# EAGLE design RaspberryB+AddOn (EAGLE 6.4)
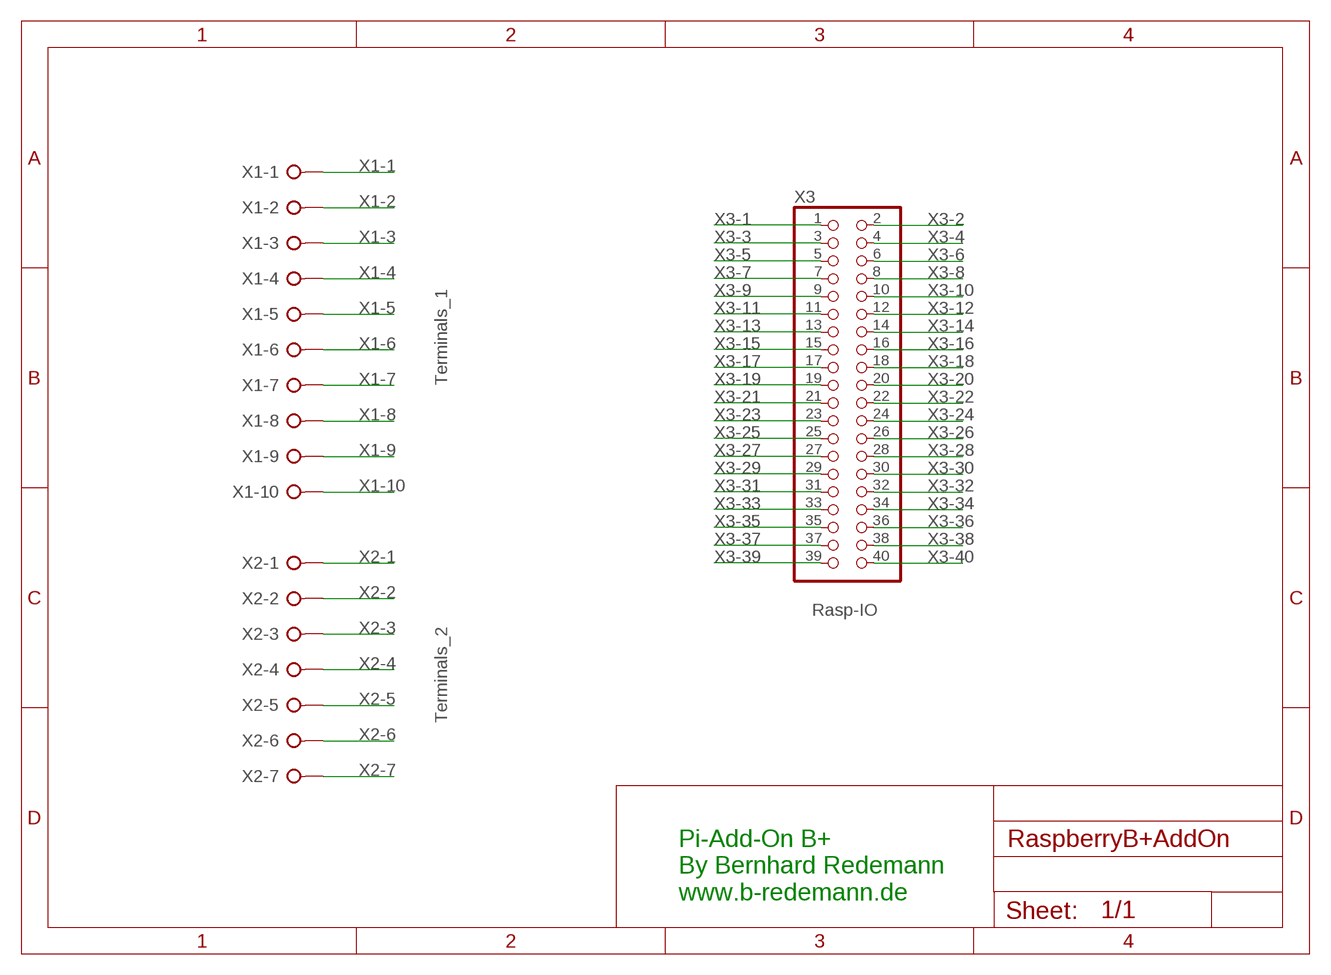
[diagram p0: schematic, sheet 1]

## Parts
X1  Terminals_1  W237-10P  [W237-10P]
X2  Terminals_2  W237-07P  [W237-7P]
X3  Rasp-IO  PINHD-2X20  [2X20]

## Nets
X1-1: X1.1
X1-2: X1.2
X1-3: X1.3
X1-4: X1.4
X1-5: X1.5
X1-6: X1.6
X1-7: X1.7
X1-8: X1.8
X1-9: X1.9
X1-10: X1.10
X2-1: X2.1
X2-2: X2.2
X2-3: X2.3
X2-4: X2.4
X2-5: X2.5
X2-6: X2.6
X2-7: X2.7
X3-1: X3.1
X3-2: X3.2
X3-3: X3.3
X3-4: X3.4
X3-5: X3.5
X3-6: X3.6
X3-7: X3.7
X3-8: X3.8
X3-9: X3.9
X3-10: X3.10
X3-11: X3.11
X3-12: X3.12
X3-13: X3.13
X3-14: X3.14
X3-15: X3.15
X3-16: X3.16
X3-17: X3.17
X3-18: X3.18
X3-19: X3.19
X3-20: X3.20
X3-21: X3.21
X3-22: X3.22
X3-23: X3.23
X3-24: X3.24
X3-25: X3.25
X3-26: X3.26
X3-27: X3.27
X3-28: X3.28
X3-29: X3.29
X3-30: X3.30
X3-31: X3.31
X3-32: X3.32
X3-33: X3.33
X3-34: X3.34
X3-35: X3.35
X3-36: X3.36
X3-37: X3.37
X3-38: X3.38
X3-39: X3.39
X3-40: X3.40

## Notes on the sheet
- Pi-Add-On B+
  By Bernhard Redemann
  www.b-redemann.de

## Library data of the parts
X1 = con-wago-508:W237-10P: WAGO SREW CLAMP; OC_FARNELL: unknown; OC_NEWARK: unknown
X2 = con-wago-508:W237-07P: WAGO SREW CLAMP; OC_FARNELL: unknown; OC_NEWARK: unknown
X3 = pinhead:PINHD-2X20: PIN HEADER

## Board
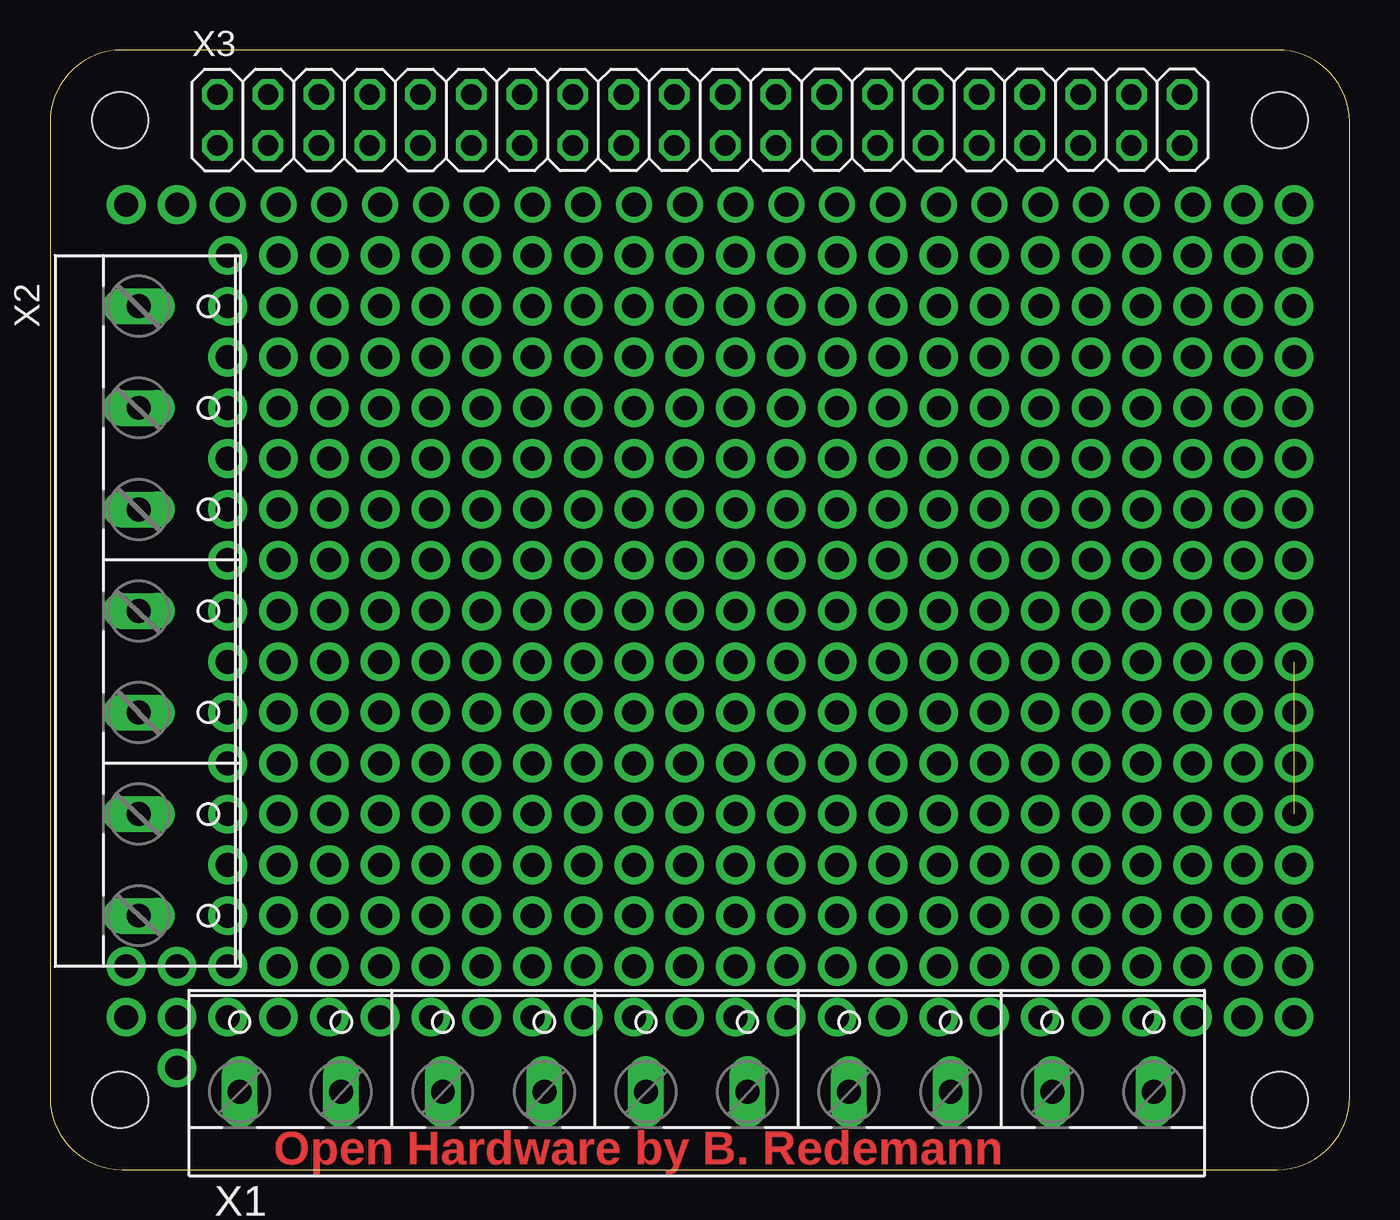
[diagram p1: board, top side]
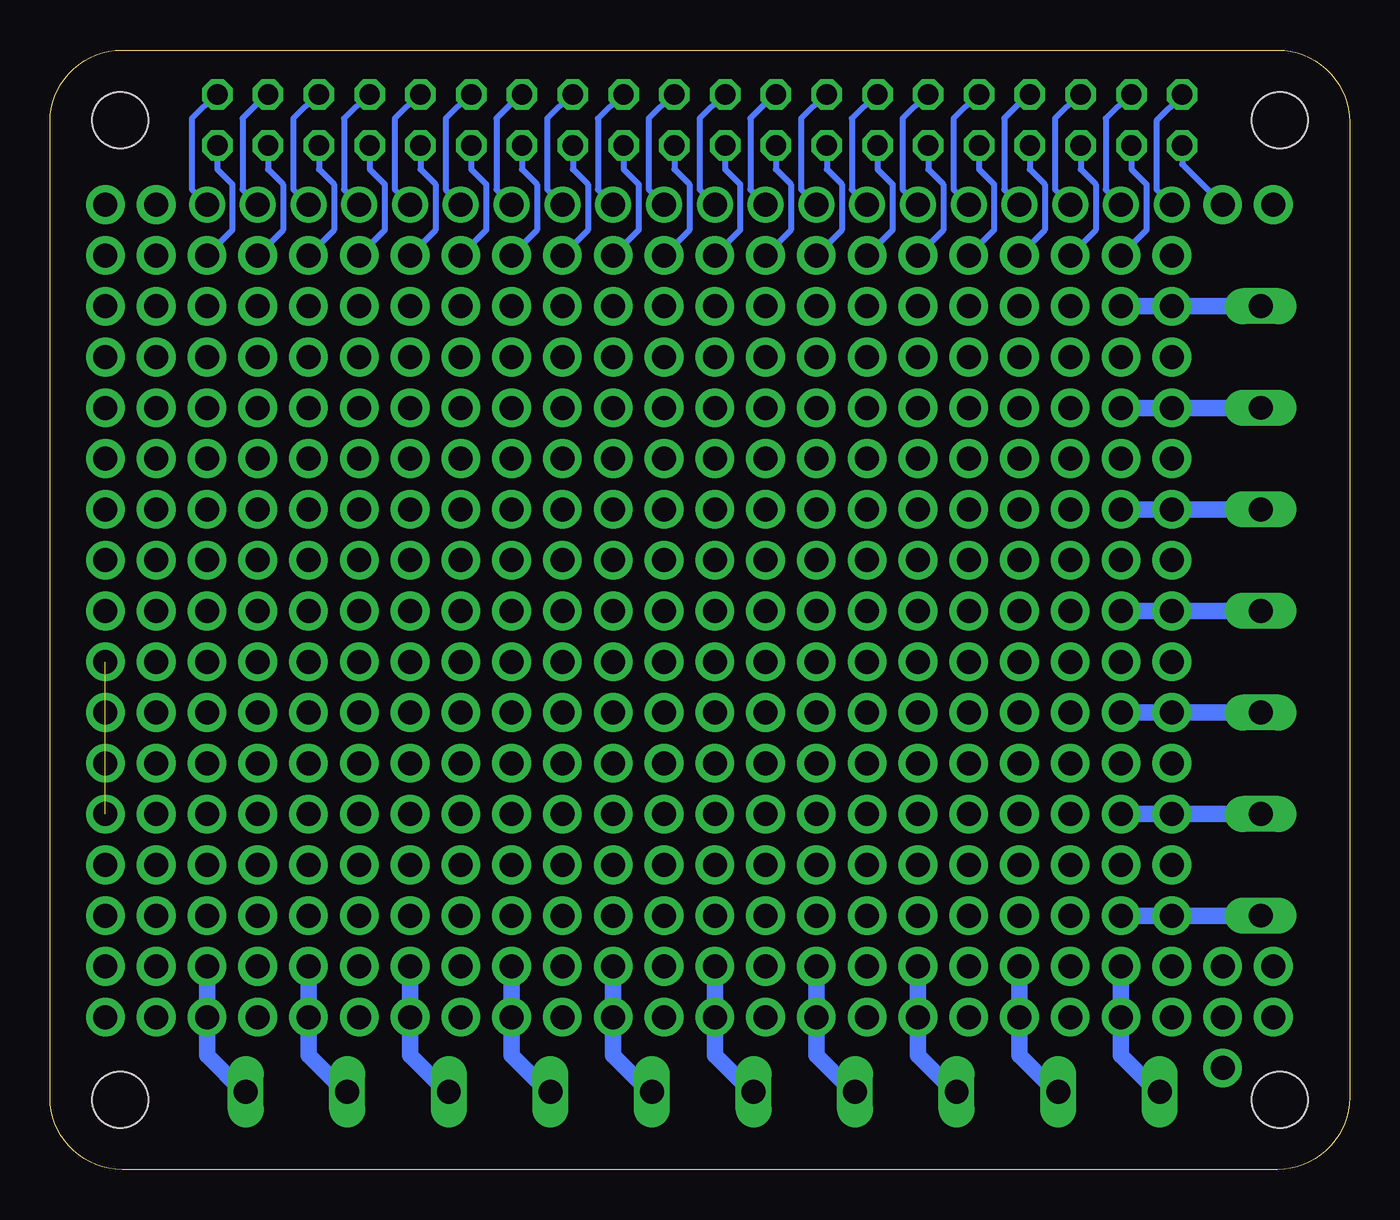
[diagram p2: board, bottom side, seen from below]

Size 65 x 56 mm. Coordinates in mm from the lower left corner, seen from the top.
Outline: 61.39,56 3.61,56 arc90 0,52.39 0,3.61 arc90 3.61,0 61.39,0 arc90 65,3.61 65,52.39 arc90 61.39,56
Copper layers (1*16): Top 0.035mm / dielectric 1.5mm / Bottom 0.035mm
Design rules "default": minimum track width 10mil, minimum drill 24mil, track to track 8mil, track to pad 8mil, pad to pad 8mil, via to via 8mil, smd to smd 8mil, copper to edge 40mil, drill to drill 8mil, minimum pad ring 10mil, minimum via ring 8mil, stop-mask expansion 4mil, vias tented up to drill 0mil, thermal gap 10mil
Holes 2.8 mm at 3.5,3.5 3.5,52.5 61.5,3.5 61.5,52.5

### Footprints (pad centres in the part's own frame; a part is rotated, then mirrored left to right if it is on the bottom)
W237-10P = drill 1.194 long: 1 -22.86,-0.635; 2 -17.78,-0.635; 3 -12.7,-0.635; 4 -7.62,-0.635; 5 -2.54,-0.635; 6 2.54,-0.635; 7 7.62,-0.635; 8 12.7,-0.635; 9 17.78,-0.635; 10 22.86,-0.635
W237-7P = drill 1.194 long: 1 -15.24,-0.635; 2 -10.16,-0.635; 3 -5.08,-0.635; 4 0,-0.635; 5 5.08,-0.635; 6 10.16,-0.635; 7 15.24,-0.635
2X20 = drill 1.016 octagon: 1 -24.13,-1.27; 2 -24.13,1.27; 3 -21.59,-1.27; 4 -21.59,1.27; 5 -19.05,-1.27; 6 -19.05,1.27; 7 -16.51,-1.27; 8 -16.51,1.27; 9 -13.97,-1.27; 10 -13.97,1.27; 11 -11.43,-1.27; 12 -11.43,1.27; 13 -8.89,-1.27; 14 -8.89,1.27; 15 -6.35,-1.27; 16 -6.35,1.27; 17 -3.81,-1.27; 18 -3.81,1.27; 19 -1.27,-1.27; 20 -1.27,1.27; 21 1.27,-1.27; 22 1.27,1.27; 23 3.81,-1.27; 24 3.81,1.27; 25 6.35,-1.27; 26 6.35,1.27; 27 8.89,-1.27; 28 8.89,1.27; 29 11.43,-1.27; 30 11.43,1.27; 31 13.97,-1.27; 32 13.97,1.27; 33 16.51,-1.27; 34 16.51,1.27; 35 19.05,-1.27; 36 19.05,1.27; 37 21.59,-1.27; 38 21.59,1.27; 39 24.13,-1.27; 40 24.13,1.27

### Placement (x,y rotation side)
X1  32.35,4.53 0 top
X2  5.08,27.94 270 top
X3  32.5,52.5 0 top

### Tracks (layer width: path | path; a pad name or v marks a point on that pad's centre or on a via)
N$1  (via drill 1.2 pad 1.93)
  other vias: 3.81,48.26
N$23  (via drill 1.2 pad 1.93)
  other vias: 59.69,48.26
N$24  (via drill 1.2 pad 1.93)
  other vias: 62.23,48.26
N$25  (via drill 1.2 pad 1.93)
  other vias: 62.23,45.72
N$26  (via drill 1.2 pad 1.93)
  other vias: 59.69,45.72
N$54  (via drill 1.2 pad 1.93)
  other vias: 8.89,45.72
N$55  (via drill 1.2 pad 1.93)
  other vias: 13.97,43.18
N$56  (via drill 1.2 pad 1.93)
  other vias: 16.51,43.18
N$57  (via drill 1.2 pad 1.93)
  other vias: 19.05,43.18
N$58  (via drill 1.2 pad 1.93)
  other vias: 21.59,43.18
N$59  (via drill 1.2 pad 1.93)
  other vias: 24.13,43.18
N$60  (via drill 1.2 pad 1.93)
  other vias: 26.67,43.18
N$61  (via drill 1.2 pad 1.93)
  other vias: 29.21,43.18
N$62  (via drill 1.2 pad 1.93)
  other vias: 31.75,43.18
N$63  (via drill 1.2 pad 1.93)
  other vias: 34.29,43.18
N$64  (via drill 1.2 pad 1.93)
  other vias: 36.83,43.18
N$65  (via drill 1.2 pad 1.93)
  other vias: 39.37,43.18
N$66  (via drill 1.2 pad 1.93)
  other vias: 41.91,43.18
N$67  (via drill 1.2 pad 1.93)
  other vias: 44.45,43.18
N$68  (via drill 1.2 pad 1.93)
  other vias: 46.99,43.18
N$69  (via drill 1.2 pad 1.93)
  other vias: 49.53,43.18
N$70  (via drill 1.2 pad 1.93)
  other vias: 52.07,43.18
N$71  (via drill 1.2 pad 1.93)
  other vias: 54.61,43.18
N$72  (via drill 1.2 pad 1.93)
  other vias: 57.15,43.18
N$73  (via drill 1.2 pad 1.93)
  other vias: 59.69,43.18
N$74  (via drill 1.2 pad 1.93)
  other vias: 62.23,43.18
N$75  (via drill 1.2 pad 1.93)
  other vias: 62.23,40.64
N$76  (via drill 1.2 pad 1.93)
  other vias: 62.23,38.1
N$77  (via drill 1.2 pad 1.93)
  other vias: 59.69,40.64
N$78  (via drill 1.2 pad 1.93)
  other vias: 59.69,38.1
N$79  (via drill 1.2 pad 1.93)
  other vias: 57.15,40.64
N$80  (via drill 1.2 pad 1.93)
  other vias: 57.15,38.1
N$81  (via drill 1.2 pad 1.93)
  other vias: 54.61,40.64
N$82  (via drill 1.2 pad 1.93)
  other vias: 54.61,38.1
N$83  (via drill 1.2 pad 1.93)
  other vias: 52.07,40.64
N$84  (via drill 1.2 pad 1.93)
  other vias: 52.07,38.1
N$85  (via drill 1.2 pad 1.93)
  other vias: 49.53,40.64
N$86  (via drill 1.2 pad 1.93)
  other vias: 49.53,38.1
N$87  (via drill 1.2 pad 1.93)
  other vias: 46.99,40.64
N$88  (via drill 1.2 pad 1.93)
  other vias: 46.99,38.1
N$89  (via drill 1.2 pad 1.93)
  other vias: 44.45,40.64
N$90  (via drill 1.2 pad 1.93)
  other vias: 44.45,38.1
N$91  (via drill 1.2 pad 1.93)
  other vias: 41.91,40.64
N$92  (via drill 1.2 pad 1.93)
  other vias: 41.91,38.1
N$93  (via drill 1.2 pad 1.93)
  other vias: 39.37,40.64
N$94  (via drill 1.2 pad 1.93)
  other vias: 39.37,38.1
N$95  (via drill 1.2 pad 1.93)
  other vias: 36.83,40.64
N$96  (via drill 1.2 pad 1.93)
  other vias: 36.83,38.1
N$97  (via drill 1.2 pad 1.93)
  other vias: 34.29,40.64
N$98  (via drill 1.2 pad 1.93)
  other vias: 34.29,38.1
N$99  (via drill 1.2 pad 1.93)
  other vias: 31.75,40.64
N$100  (via drill 1.2 pad 1.93)
  other vias: 31.75,38.1
N$101  (via drill 1.2 pad 1.93)
  other vias: 29.21,40.64
N$102  (via drill 1.2 pad 1.93)
  other vias: 29.21,38.1
N$103  (via drill 1.2 pad 1.93)
  other vias: 26.67,40.64
N$104  (via drill 1.2 pad 1.93)
  other vias: 26.67,38.1
N$105  (via drill 1.2 pad 1.93)
  other vias: 24.13,40.64
N$106  (via drill 1.2 pad 1.93)
  other vias: 24.13,38.1
N$107  (via drill 1.2 pad 1.93)
  other vias: 21.59,40.64
N$108  (via drill 1.2 pad 1.93)
  other vias: 21.59,38.1
N$109  (via drill 1.2 pad 1.93)
  other vias: 19.05,40.64
N$110  (via drill 1.2 pad 1.93)
  other vias: 19.05,38.1
N$111  (via drill 1.2 pad 1.93)
  other vias: 16.51,40.64
N$112  (via drill 1.2 pad 1.93)
  other vias: 16.51,38.1
N$113  (via drill 1.2 pad 1.93)
  other vias: 13.97,40.64
N$114  (via drill 1.2 pad 1.93)
  other vias: 13.97,38.1
N$116  (via drill 1.2 pad 1.93)
  other vias: 8.89,40.64
N$118  (via drill 1.2 pad 1.93)
  other vias: 11.43,40.64
N$125  (via drill 1.2 pad 1.93)
  other vias: 13.97,35.56
N$126  (via drill 1.2 pad 1.93)
  other vias: 16.51,35.56
N$127  (via drill 1.2 pad 1.93)
  other vias: 19.05,35.56
N$128  (via drill 1.2 pad 1.93)
  other vias: 21.59,35.56
N$129  (via drill 1.2 pad 1.93)
  other vias: 24.13,35.56
N$130  (via drill 1.2 pad 1.93)
  other vias: 26.67,35.56
N$131  (via drill 1.2 pad 1.93)
  other vias: 29.21,35.56
N$132  (via drill 1.2 pad 1.93)
  other vias: 31.75,35.56
N$133  (via drill 1.2 pad 1.93)
  other vias: 34.29,35.56
N$134  (via drill 1.2 pad 1.93)
  other vias: 36.83,35.56
N$135  (via drill 1.2 pad 1.93)
  other vias: 39.37,35.56
N$136  (via drill 1.2 pad 1.93)
  other vias: 41.91,35.56
N$137  (via drill 1.2 pad 1.93)
  other vias: 44.45,35.56
N$138  (via drill 1.2 pad 1.93)
  other vias: 46.99,35.56
N$139  (via drill 1.2 pad 1.93)
  other vias: 49.53,35.56
N$140  (via drill 1.2 pad 1.93)
  other vias: 52.07,35.56
N$141  (via drill 1.2 pad 1.93)
  other vias: 54.61,35.56
N$142  (via drill 1.2 pad 1.93)
  other vias: 57.15,35.56
N$143  (via drill 1.2 pad 1.93)
  other vias: 59.69,35.56
N$144  (via drill 1.2 pad 1.93)
  other vias: 62.23,35.56
N$145  (via drill 1.2 pad 1.93)
  other vias: 62.23,33.02
N$146  (via drill 1.2 pad 1.93)
  other vias: 62.23,30.48
N$147  (via drill 1.2 pad 1.93)
  other vias: 62.23,27.94
N$150  (via drill 1.2 pad 1.93)
  other vias: 8.89,35.56
N$151  (via drill 1.2 pad 1.93)
  other vias: 11.43,35.56
N$152  (via drill 1.2 pad 1.93)
  other vias: 13.97,33.02
N$153  (via drill 1.2 pad 1.93)
  other vias: 16.51,33.02
N$154  (via drill 1.2 pad 1.93)
  other vias: 19.05,33.02
N$155  (via drill 1.2 pad 1.93)
  other vias: 21.59,33.02
N$156  (via drill 1.2 pad 1.93)
  other vias: 24.13,33.02
N$157  (via drill 1.2 pad 1.93)
  other vias: 26.67,33.02
N$158  (via drill 1.2 pad 1.93)
  other vias: 29.21,33.02
N$159  (via drill 1.2 pad 1.93)
  other vias: 31.75,33.02
N$160  (via drill 1.2 pad 1.93)
  other vias: 34.29,33.02
N$161  (via drill 1.2 pad 1.93)
  other vias: 36.83,33.02
N$162  (via drill 1.2 pad 1.93)
  other vias: 39.37,33.02
N$163  (via drill 1.2 pad 1.93)
  other vias: 41.91,33.02
N$164  (via drill 1.2 pad 1.93)
  other vias: 44.45,33.02
N$165  (via drill 1.2 pad 1.93)
  other vias: 46.99,33.02
N$166  (via drill 1.2 pad 1.93)
  other vias: 49.53,33.02
N$167  (via drill 1.2 pad 1.93)
  other vias: 52.07,33.02
N$168  (via drill 1.2 pad 1.93)
  other vias: 54.61,33.02
N$169  (via drill 1.2 pad 1.93)
  other vias: 57.15,33.02
N$170  (via drill 1.2 pad 1.93)
  other vias: 59.69,33.02
N$171  (via drill 1.2 pad 1.93)
  other vias: 59.69,30.48
N$172  (via drill 1.2 pad 1.93)
  other vias: 57.15,30.48
N$173  (via drill 1.2 pad 1.93)
  other vias: 54.61,30.48
N$174  (via drill 1.2 pad 1.93)
  other vias: 52.07,30.48
N$175  (via drill 1.2 pad 1.93)
  other vias: 49.53,30.48
N$176  (via drill 1.2 pad 1.93)
  other vias: 46.99,30.48
N$177  (via drill 1.2 pad 1.93)
  other vias: 44.45,30.48
N$178  (via drill 1.2 pad 1.93)
  other vias: 41.91,30.48
N$179  (via drill 1.2 pad 1.93)
  other vias: 39.37,30.48
N$180  (via drill 1.2 pad 1.93)
  other vias: 36.83,30.48
N$181  (via drill 1.2 pad 1.93)
  other vias: 34.29,30.48
N$182  (via drill 1.2 pad 1.93)
  other vias: 31.75,30.48
N$183  (via drill 1.2 pad 1.93)
  other vias: 29.21,30.48
N$184  (via drill 1.2 pad 1.93)
  other vias: 26.67,30.48
N$185  (via drill 1.2 pad 1.93)
  other vias: 24.13,30.48
N$186  (via drill 1.2 pad 1.93)
  other vias: 21.59,30.48
N$187  (via drill 1.2 pad 1.93)
  other vias: 19.05,30.48
N$188  (via drill 1.2 pad 1.93)
  other vias: 16.51,30.48
N$189  (via drill 1.2 pad 1.93)
  other vias: 13.97,30.48
N$198  (via drill 1.2 pad 1.93)
  other vias: 8.89,30.48
N$199  (via drill 1.2 pad 1.93)
  other vias: 11.43,30.48
N$200  (via drill 1.2 pad 1.93)
  other vias: 13.97,27.94
N$201  (via drill 1.2 pad 1.93)
  other vias: 16.51,27.94
N$202  (via drill 1.2 pad 1.93)
  other vias: 19.05,27.94
N$203  (via drill 1.2 pad 1.93)
  other vias: 21.59,27.94
N$204  (via drill 1.2 pad 1.93)
  other vias: 24.13,27.94
N$205  (via drill 1.2 pad 1.93)
  other vias: 26.67,27.94
N$206  (via drill 1.2 pad 1.93)
  other vias: 29.21,27.94
N$207  (via drill 1.2 pad 1.93)
  other vias: 31.75,27.94
N$208  (via drill 1.2 pad 1.93)
  other vias: 34.29,27.94
N$209  (via drill 1.2 pad 1.93)
  other vias: 36.83,27.94
N$210  (via drill 1.2 pad 1.93)
  other vias: 39.37,27.94
N$211  (via drill 1.2 pad 1.93)
  other vias: 41.91,27.94
N$212  (via drill 1.2 pad 1.93)
  other vias: 44.45,27.94
N$213  (via drill 1.2 pad 1.93)
  other vias: 46.99,27.94
N$214  (via drill 1.2 pad 1.93)
  other vias: 49.53,27.94
N$215  (via drill 1.2 pad 1.93)
  other vias: 52.07,27.94
N$216  (via drill 1.2 pad 1.93)
  other vias: 54.61,27.94
N$217  (via drill 1.2 pad 1.93)
  other vias: 57.15,27.94
N$218  (via drill 1.2 pad 1.93)
  other vias: 59.69,27.94
N$219  (via drill 1.2 pad 1.93)
  other vias: 59.69,25.4
N$220  (via drill 1.2 pad 1.93)
  other vias: 59.69,22.86
N$221  (via drill 1.2 pad 1.93)
  other vias: 57.15,25.4
N$222  (via drill 1.2 pad 1.93)
  other vias: 57.15,22.86
N$223  (via drill 1.2 pad 1.93)
  other vias: 54.61,25.4
N$224  (via drill 1.2 pad 1.93)
  other vias: 54.61,22.86
N$225  (via drill 1.2 pad 1.93)
  other vias: 52.07,25.4
N$226  (via drill 1.2 pad 1.93)
  other vias: 52.07,22.86
N$227  (via drill 1.2 pad 1.93)
  other vias: 49.53,25.4
N$228  (via drill 1.2 pad 1.93)
  other vias: 49.53,22.86
N$229  (via drill 1.2 pad 1.93)
  other vias: 46.99,25.4
N$230  (via drill 1.2 pad 1.93)
  other vias: 46.99,22.86
N$231  (via drill 1.2 pad 1.93)
  other vias: 44.45,25.4
N$232  (via drill 1.2 pad 1.93)
  other vias: 44.45,22.86
N$233  (via drill 1.2 pad 1.93)
  other vias: 41.91,25.4
N$234  (via drill 1.2 pad 1.93)
  other vias: 41.91,22.86
N$235  (via drill 1.2 pad 1.93)
  other vias: 39.37,25.4
N$236  (via drill 1.2 pad 1.93)
  other vias: 39.37,22.86
N$237  (via drill 1.2 pad 1.93)
  other vias: 36.83,25.4
N$238  (via drill 1.2 pad 1.93)
  other vias: 36.83,22.86
N$239  (via drill 1.2 pad 1.93)
  other vias: 34.29,25.4
N$240  (via drill 1.2 pad 1.93)
  other vias: 34.29,22.86
N$241  (via drill 1.2 pad 1.93)
  other vias: 31.75,25.4
N$242  (via drill 1.2 pad 1.93)
  other vias: 31.75,22.86
N$243  (via drill 1.2 pad 1.93)
  other vias: 29.21,25.4
N$244  (via drill 1.2 pad 1.93)
  other vias: 29.21,22.86
N$245  (via drill 1.2 pad 1.93)
  other vias: 26.67,25.4
N$246  (via drill 1.2 pad 1.93)
  other vias: 26.67,22.86
N$247  (via drill 1.2 pad 1.93)
  other vias: 24.13,25.4
N$248  (via drill 1.2 pad 1.93)
  other vias: 24.13,22.86
N$249  (via drill 1.2 pad 1.93)
  other vias: 21.59,25.4
N$250  (via drill 1.2 pad 1.93)
  other vias: 21.59,22.86
N$251  (via drill 1.2 pad 1.93)
  other vias: 19.05,25.4
N$252  (via drill 1.2 pad 1.93)
  other vias: 19.05,22.86
N$253  (via drill 1.2 pad 1.93)
  other vias: 16.51,25.4
N$254  (via drill 1.2 pad 1.93)
  other vias: 16.51,22.86
N$255  (via drill 1.2 pad 1.93)
  other vias: 13.97,25.4
N$256  (via drill 1.2 pad 1.93)
  other vias: 13.97,22.86
N$258  (via drill 1.2 pad 1.93)
  other vias: 11.43,25.4
N$260  (via drill 1.2 pad 1.93)
  other vias: 8.89,25.4
N$267  (via drill 1.2 pad 1.93)
  other vias: 13.97,20.32
N$268  (via drill 1.2 pad 1.93)
  other vias: 16.51,20.32
N$269  (via drill 1.2 pad 1.93)
  other vias: 19.05,20.32
N$270  (via drill 1.2 pad 1.93)
  other vias: 21.59,20.32
N$271  (via drill 1.2 pad 1.93)
  other vias: 24.13,20.32
N$272  (via drill 1.2 pad 1.93)
  other vias: 26.67,20.32
N$273  (via drill 1.2 pad 1.93)
  other vias: 29.21,20.32
N$274  (via drill 1.2 pad 1.93)
  other vias: 31.75,20.32
N$275  (via drill 1.2 pad 1.93)
  other vias: 34.29,20.32
N$276  (via drill 1.2 pad 1.93)
  other vias: 36.83,20.32
N$277  (via drill 1.2 pad 1.93)
  other vias: 39.37,20.32
N$278  (via drill 1.2 pad 1.93)
  other vias: 41.91,20.32
N$279  (via drill 1.2 pad 1.93)
  other vias: 44.45,20.32
N$280  (via drill 1.2 pad 1.93)
  other vias: 46.99,20.32
N$281  (via drill 1.2 pad 1.93)
  other vias: 49.53,20.32
N$282  (via drill 1.2 pad 1.93)
  other vias: 52.07,20.32
N$283  (via drill 1.2 pad 1.93)
  other vias: 54.61,20.32
N$284  (via drill 1.2 pad 1.93)
  other vias: 57.15,20.32
N$285  (via drill 1.2 pad 1.93)
  other vias: 59.69,20.32
N$286  (via drill 1.2 pad 1.93)  (3 unrouted)
  other vias: 62.23,17.78 62.23,20.32 62.23,22.86 62.23,25.4
N$287  (via drill 1.2 pad 1.93)
  other vias: 62.23,15.24
N$288  (via drill 1.2 pad 1.93)
  other vias: 62.23,12.7
N$291  (via drill 1.2 pad 1.93)
  other vias: 8.89,20.32
N$292  (via drill 1.2 pad 1.93)
  other vias: 11.43,20.32
N$293  (via drill 1.2 pad 1.93)
  other vias: 13.97,17.78
N$294  (via drill 1.2 pad 1.93)
  other vias: 16.51,17.78
N$295  (via drill 1.2 pad 1.93)
  other vias: 19.05,17.78
N$296  (via drill 1.2 pad 1.93)
  other vias: 21.59,17.78
N$297  (via drill 1.2 pad 1.93)
  other vias: 24.13,17.78
N$298  (via drill 1.2 pad 1.93)
  other vias: 26.67,17.78
N$299  (via drill 1.2 pad 1.93)
  other vias: 29.21,17.78
N$300  (via drill 1.2 pad 1.93)
  other vias: 31.75,17.78
N$301  (via drill 1.2 pad 1.93)
  other vias: 34.29,17.78
N$302  (via drill 1.2 pad 1.93)
  other vias: 36.83,17.78
N$303  (via drill 1.2 pad 1.93)
  other vias: 39.37,17.78
N$304  (via drill 1.2 pad 1.93)
  other vias: 41.91,17.78
N$305  (via drill 1.2 pad 1.93)
  other vias: 44.45,17.78
N$306  (via drill 1.2 pad 1.93)
  other vias: 46.99,17.78
N$307  (via drill 1.2 pad 1.93)
  other vias: 49.53,17.78
N$308  (via drill 1.2 pad 1.93)
  other vias: 52.07,17.78
N$309  (via drill 1.2 pad 1.93)
  other vias: 54.61,17.78
N$310  (via drill 1.2 pad 1.93)
  other vias: 57.15,17.78
N$311  (via drill 1.2 pad 1.93)
  other vias: 59.69,17.78
N$312  (via drill 1.2 pad 1.93)
  other vias: 59.69,15.24
N$313  (via drill 1.2 pad 1.93)
  other vias: 57.15,15.24
N$314  (via drill 1.2 pad 1.93)
  other vias: 54.61,15.24
N$315  (via drill 1.2 pad 1.93)
  other vias: 52.07,15.24
N$316  (via drill 1.2 pad 1.93)
  other vias: 49.53,15.24
N$317  (via drill 1.2 pad 1.93)
  other vias: 46.99,15.24
N$318  (via drill 1.2 pad 1.93)
  other vias: 44.45,15.24
N$319  (via drill 1.2 pad 1.93)
  other vias: 41.91,15.24
N$320  (via drill 1.2 pad 1.93)
  other vias: 39.37,15.24
N$321  (via drill 1.2 pad 1.93)
  other vias: 36.83,15.24
N$322  (via drill 1.2 pad 1.93)
  other vias: 34.29,15.24
N$323  (via drill 1.2 pad 1.93)
  other vias: 31.75,15.24
N$324  (via drill 1.2 pad 1.93)
  other vias: 29.21,15.24
N$325  (via drill 1.2 pad 1.93)
  other vias: 26.67,15.24
N$326  (via drill 1.2 pad 1.93)
  other vias: 24.13,15.24
N$327  (via drill 1.2 pad 1.93)
  other vias: 21.59,15.24
N$328  (via drill 1.2 pad 1.93)
  other vias: 19.05,15.24
N$329  (via drill 1.2 pad 1.93)
  other vias: 16.51,15.24
N$330  (via drill 1.2 pad 1.93)
  other vias: 13.97,15.24
N$336  (via drill 1.2 pad 1.93)
  other vias: 3.81,10.16
N$337  (via drill 1.2 pad 1.93)
  other vias: 6.35,10.16
N$339  (via drill 1.2 pad 1.93)
  other vias: 11.43,15.24
N$340  (via drill 1.2 pad 1.93)
  other vias: 8.89,15.24
N$341  (via drill 1.2 pad 1.93)
  other vias: 13.97,12.7
N$342  (via drill 1.2 pad 1.93)
  other vias: 16.51,12.7
N$343  (via drill 1.2 pad 1.93)
  other vias: 19.05,12.7
N$344  (via drill 1.2 pad 1.93)
  other vias: 21.59,12.7
N$345  (via drill 1.2 pad 1.93)
  other vias: 24.13,12.7
N$346  (via drill 1.2 pad 1.93)
  other vias: 26.67,12.7
N$347  (via drill 1.2 pad 1.93)
  other vias: 29.21,12.7
N$348  (via drill 1.2 pad 1.93)
  other vias: 31.75,12.7
N$349  (via drill 1.2 pad 1.93)
  other vias: 34.29,12.7
N$350  (via drill 1.2 pad 1.93)
  other vias: 36.83,12.7
N$351  (via drill 1.2 pad 1.93)
  other vias: 39.37,12.7
N$352  (via drill 1.2 pad 1.93)
  other vias: 41.91,12.7
N$353  (via drill 1.2 pad 1.93)
  other vias: 44.45,12.7
N$354  (via drill 1.2 pad 1.93)
  other vias: 46.99,12.7
N$355  (via drill 1.2 pad 1.93)
  other vias: 49.53,12.7
N$356  (via drill 1.2 pad 1.93)
  other vias: 52.07,12.7
N$357  (via drill 1.2 pad 1.93)
  other vias: 54.61,12.7
N$358  (via drill 1.2 pad 1.93)
  other vias: 57.15,12.7
N$359  (via drill 1.2 pad 1.93)
  other vias: 59.69,12.7
N$360  (via drill 1.2 pad 1.93)
  other vias: 59.69,10.16
N$361  (via drill 1.2 pad 1.93)
  other vias: 59.69,7.62
N$364  (via drill 1.2 pad 1.93)
  other vias: 54.61,10.16
N$365  (via drill 1.2 pad 1.93)
  other vias: 54.61,7.62
N$368  (via drill 1.2 pad 1.93)
  other vias: 49.53,10.16
N$369  (via drill 1.2 pad 1.93)
  other vias: 49.53,7.62
N$372  (via drill 1.2 pad 1.93)
  other vias: 44.45,10.16
N$373  (via drill 1.2 pad 1.93)
  other vias: 44.45,7.62
N$376  (via drill 1.2 pad 1.93)
  other vias: 39.37,10.16
N$377  (via drill 1.2 pad 1.93)
  other vias: 39.37,7.62
N$380  (via drill 1.2 pad 1.93)
  other vias: 34.29,10.16
N$381  (via drill 1.2 pad 1.93)
  other vias: 34.29,7.62
N$384  (via drill 1.2 pad 1.93)
  other vias: 29.21,10.16
N$385  (via drill 1.2 pad 1.93)
  other vias: 29.21,7.62
N$388  (via drill 1.2 pad 1.93)
  other vias: 24.13,10.16
N$389  (via drill 1.2 pad 1.93)
  other vias: 24.13,7.62
N$392  (via drill 1.2 pad 1.93)
  other vias: 19.05,10.16
N$393  (via drill 1.2 pad 1.93)
  other vias: 19.05,7.62
N$396  (via drill 1.2 pad 1.93)
  other vias: 13.97,10.16
N$397  (via drill 1.2 pad 1.93)
  other vias: 13.97,7.62
N$400  (via drill 1.2 pad 1.93)
  other vias: 8.89,10.16
N$401  (via drill 1.2 pad 1.93)
  other vias: 8.89,7.62
N$402  (via drill 1.2 pad 1.93)
  other vias: 6.35,7.62
N$403  (via drill 1.2 pad 1.93)
  other vias: 3.81,7.62
N$404  (via drill 1.2 pad 1.93)
  other vias: 62.23,7.62
N$405  (via drill 1.2 pad 1.93)
  other vias: 6.35,5.08
N$426  (via drill 1.2 pad 1.93)
  other vias: 62.23,10.16
X1-1  (via drill 1.2 pad 1.93)
  Bottom 0.813: X1.1 9.61,3.89 11.43,5.71 v11.43,7.62 v11.43,10.16
X1-2  (via drill 1.2 pad 1.93)
  Bottom 0.813: X1.2 14.69,3.89 16.51,5.71 v16.51,7.62 v16.51,10.16
X1-3  (via drill 1.2 pad 1.93)
  Bottom 0.813: X1.3 19.77,3.89 21.59,5.71 v21.59,7.62 v21.59,10.16
X1-4  (via drill 1.2 pad 1.93)
  Bottom 0.813: X1.4 24.84,3.89 26.67,5.71 v26.67,7.62 v26.67,10.16
X1-5  (via drill 1.2 pad 1.93)
  Bottom 0.813: X1.5 29.93,3.89 31.75,5.71 v31.75,7.62 v31.75,10.16
X1-6  (via drill 1.2 pad 1.93)
  Bottom 0.813: X1.6 35.01,3.89 36.83,5.71 v36.83,7.62 v36.83,10.16
X1-7  (via drill 1.2 pad 1.93)
  Bottom 0.813: X1.7 40.09,3.89 41.91,5.71 v41.91,7.62 v41.91,10.16
X1-8  (via drill 1.2 pad 1.93)
  Bottom 0.813: X1.8 45.16,3.89 46.99,5.71 v46.99,7.62 v46.99,10.16
X1-9  (via drill 1.2 pad 1.93)
  Bottom 0.813: X1.9 50.24,3.89 52.07,5.71 v52.07,7.62 v52.07,10.16
X1-10  (via drill 1.2 pad 1.93)
  Bottom 0.813: X1.10 55.33,3.89 57.15,5.71 v57.15,7.62 v57.15,10.16
X2-1  (via drill 1.2 pad 1.93)
  Bottom 0.813: v11.43,43.18 v8.89,43.18 X2.1
X2-2  (via drill 1.2 pad 1.93)
  Bottom 0.813: v11.43,38.1 v8.89,38.1 X2.2
X2-3  (via drill 1.2 pad 1.93)
  Bottom 0.813: v11.43,33.02 v8.89,33.02 X2.3
X2-4  (via drill 1.2 pad 1.93)
  Bottom 0.813: v11.43,27.94 v8.89,27.94 X2.4
X2-5  (via drill 1.2 pad 1.93)
  Bottom 0.813: v11.43,22.86 v8.89,22.86 X2.5
X2-6  (via drill 1.2 pad 1.93)
  Bottom 0.813: v11.43,17.78 v8.89,17.78 X2.6
X2-7  (via drill 1.2 pad 1.93)
  Bottom 0.813: v11.43,12.7 v8.89,12.7 X2.7
X3-1  (via drill 1.2 pad 1.93)
  Bottom 0.305: X3.1 8.37,50.28 v6.35,48.26
X3-2  (via drill 1.2 pad 1.78)
  Bottom 0.305: X3.2 8.37,53.73 9.65,52.45 9.65,49.02 v8.89,48.26
X3-3  (via drill 1.2 pad 1.93)
  Bottom 0.305: X3.3 10.91,50.03 10.16,49.28 10.16,46.99 v11.43,45.72
X3-4  (via drill 1.2 pad 1.78)
  Bottom 0.305: X3.4 11,53.77 12.19,52.58 12.19,49.02 v11.43,48.26
X3-5  (via drill 1.2 pad 1.93)
  Bottom 0.305: X3.5 13.45,50.03 12.7,49.28 12.7,46.99 v13.97,45.72
X3-6  (via drill 1.2 pad 1.78)
  Bottom 0.305: X3.6 13.54,53.77 14.73,52.58 14.73,49.02 v13.97,48.26
X3-7  (via drill 1.2 pad 1.93)
  Bottom 0.305: X3.7 15.99,50.03 15.24,49.28 15.24,46.99 v16.51,45.72
X3-8  (via drill 1.2 pad 1.78)
  Bottom 0.305: X3.8 16.08,53.77 17.27,52.58 17.27,49.02 v16.51,48.26
X3-9  (via drill 1.2 pad 1.93)
  Bottom 0.305: X3.9 18.53,50.03 17.78,49.28 17.78,46.99 v19.05,45.72
X3-10  (via drill 1.2 pad 1.78)
  Bottom 0.305: X3.10 18.62,53.77 19.81,52.58 19.81,49.02 v19.05,48.26
X3-11  (via drill 1.2 pad 1.93)
  Bottom 0.305: X3.11 21.07,50.03 20.32,49.28 20.32,46.99 v21.59,45.72
X3-12  (via drill 1.2 pad 1.78)
  Bottom 0.305: X3.12 21.16,53.77 22.35,52.58 22.35,49.02 v21.59,48.26
X3-13  (via drill 1.2 pad 1.93)
  Bottom 0.305: X3.13 23.61,50.03 22.86,49.28 22.86,46.99 v24.13,45.72
X3-14  (via drill 1.2 pad 1.78)
  Bottom 0.305: X3.14 23.7,53.77 24.89,52.58 24.89,49.02 v24.13,48.26
X3-15  (via drill 1.2 pad 1.93)
  Bottom 0.305: X3.15 26.15,50.03 25.4,49.28 25.4,46.99 v26.67,45.72
X3-16  (via drill 1.2 pad 1.78)
  Bottom 0.305: X3.16 26.24,53.77 27.43,52.58 27.43,49.02 v26.67,48.26
X3-17  (via drill 1.2 pad 1.93)
  Bottom 0.305: X3.17 28.69,50.03 27.94,49.28 27.94,46.99 v29.21,45.72
X3-18  (via drill 1.2 pad 1.78)
  Bottom 0.305: X3.18 28.78,53.77 29.97,52.58 29.97,49.02 v29.21,48.26
X3-19  (via drill 1.2 pad 1.93)
  Bottom 0.305: X3.19 31.23,50.03 30.48,49.28 30.48,46.99 v31.75,45.72
X3-20  (via drill 1.2 pad 1.78)
  Bottom 0.305: X3.20 31.32,53.77 32.51,52.58 32.51,49.02 v31.75,48.26
X3-21  (via drill 1.2 pad 1.93)
  Bottom 0.305: X3.21 33.77,50.03 33.02,49.28 33.02,46.99 v34.29,45.72
X3-22  (via drill 1.2 pad 1.78)
  Bottom 0.305: X3.22 33.86,53.77 35.05,52.58 35.05,49.02 v34.29,48.26
X3-23  (via drill 1.2 pad 1.93)
  Bottom 0.305: X3.23 36.31,50.03 35.56,49.28 35.56,46.99 v36.83,45.72
X3-24  (via drill 1.2 pad 1.78)
  Bottom 0.305: X3.24 36.4,53.77 37.59,52.58 37.59,49.02 v36.83,48.26
X3-25  (via drill 1.2 pad 1.93)
  Bottom 0.305: X3.25 38.85,50.03 38.1,49.28 38.1,46.99 v39.37,45.72
X3-26  (via drill 1.2 pad 1.78)
  Bottom 0.305: X3.26 38.94,53.77 40.13,52.58 40.13,49.02 v39.37,48.26
X3-27  (via drill 1.2 pad 1.93)
  Bottom 0.305: X3.27 41.39,50.03 40.64,49.28 40.64,46.99 v41.91,45.72
X3-28  (via drill 1.2 pad 1.78)
  Bottom 0.305: X3.28 41.48,53.77 42.67,52.58 42.67,49.02 v41.91,48.26
X3-29  (via drill 1.2 pad 1.93)
  Bottom 0.305: X3.29 43.93,50.03 43.18,49.28 43.18,46.99 v44.45,45.72
X3-30  (via drill 1.2 pad 1.78)
  Bottom 0.305: X3.30 44.02,53.77 45.21,52.58 45.21,49.02 v44.45,48.26
X3-31  (via drill 1.2 pad 1.93)
  Bottom 0.305: X3.31 46.47,50.03 45.72,49.28 45.72,46.99 v46.99,45.72
X3-32  (via drill 1.2 pad 1.78)
  Bottom 0.305: X3.32 46.56,53.77 47.75,52.58 47.75,49.02 v46.99,48.26
X3-33  (via drill 1.2 pad 1.93)
  Bottom 0.305: X3.33 49.01,50.03 48.26,49.28 48.26,46.99 v49.53,45.72
X3-34  (via drill 1.2 pad 1.78)
  Bottom 0.305: X3.34 49.1,53.77 50.29,52.58 50.29,49.02 v49.53,48.26
X3-35  (via drill 1.2 pad 1.93)
  Bottom 0.305: X3.35 51.55,50.03 50.8,49.28 50.8,46.99 v52.07,45.72
X3-36  (via drill 1.2 pad 1.78)
  Bottom 0.305: X3.36 51.64,53.77 52.83,52.58 52.83,49.02 v52.07,48.26
X3-37  (via drill 1.2 pad 1.93)
  Bottom 0.305: X3.37 54.09,50.03 53.34,49.28 53.34,46.99 v54.61,45.72
X3-38  (via drill 1.2 pad 1.78)
  Bottom 0.305: X3.38 54.18,53.77 55.37,52.58 55.37,49.02 v54.61,48.26
X3-39  (via drill 1.2 pad 1.93)
  Bottom 0.305: X3.39 56.63,50.03 55.88,49.28 55.88,46.99 v57.15,45.72
X3-40  (via drill 1.2 pad 1.78)
  Bottom 0.305: X3.40 56.72,53.77 57.91,52.58 57.91,49.02 v57.15,48.26

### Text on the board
Top: Open Hardware by B. Redemann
